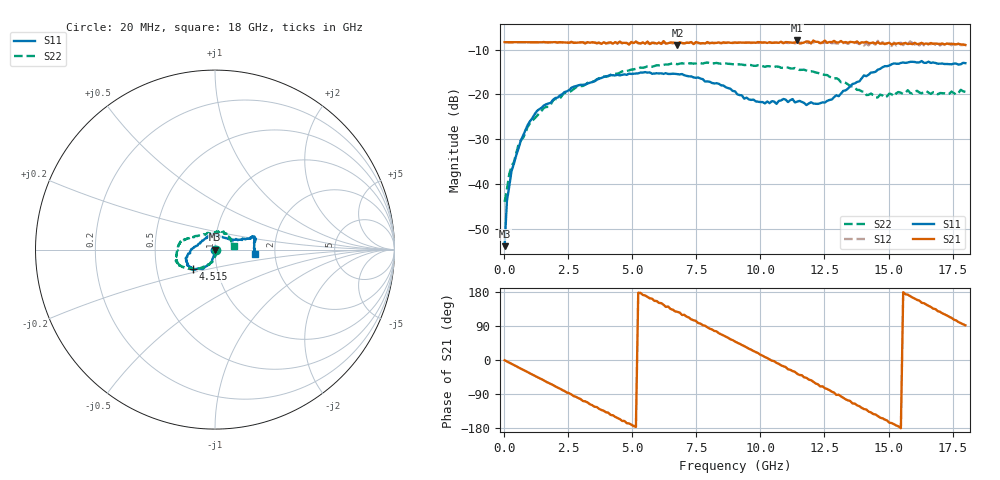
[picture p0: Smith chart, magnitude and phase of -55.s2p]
!Agilent Technologies,N5230A,US43500223,A.07.50.48
!Agilent N5230A: A.07.50.48
!Date: Monday, February 01, 2016 14:55:05
!Correction: S11(Full 2 Port(1,2))
!S21(Full 2 Port(1,2))
!S12(Full 2 Port(1,2))
!S22(Full 2 Port(1,2))
!S2P File: Measurements: S11, S21, S12, S22:
# Hz S  RI  R 50
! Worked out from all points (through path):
!   201 points, 20 MHz to 18 GHz, reference 50 ohm
!   highest |S21| = -7.93 dB at 11.44 GHz (marker M1); lowest = -9.0 dB at 6.763 GHz (marker M2)
!   group delay of S21, straight-line fit = 96.8 ps
!   lowest |S11| = -53.9 dB at 20 MHz (marker M3), VSWR 1.00, Z = 49.8 - j0.107 ohm
!   |S11| at or under -10 dB: start of sweep to end of sweep
!   |S22| runs from -44.0 to -12.9 dB; largest |S21 - S12| = 0.035
!   S11 on the Smith chart (normalised r, x): 20 MHz: 1.00, -0.00; 4.515 GHz: 0.76, -0.17; 18 GHz: 1.57, -0.08
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2e7  -0.00171 -0.00107  0.3841 -0.00414  0.3835 -0.00465  0.0063 -0.00049
1.099e8  0.000891 -0.00637  0.3827 -0.0255  0.382 -0.0262  0.00665 -0.00559
2.897e8  0.00118 -0.0139  0.3777 -0.0676  0.3772 -0.0679  0.00786 -0.0138
9.19e8  -0.00995 -0.0444  0.3258 -0.2035  0.3246 -0.2048  -0.00213 -0.0434
1.5483e9  -0.0198 -0.0726  0.2279 -0.3103  0.2256 -0.3116  -0.0149 -0.069
3.0766e9  -0.0713 -0.1064  -0.1199 -0.3631  -0.118 -0.364  -0.0748 -0.0994
4.515e9  -0.1236 -0.1068  -0.3538 -0.1585  -0.3572 -0.1582  -0.1406 -0.1042
6.0433e9  -0.1579 -0.067  -0.331 0.1856  -0.323 0.1978  -0.1912 -0.0904
6.7625e9  -0.1615 -0.0482  -0.2143 0.2825  -0.2117 0.2962  -0.2018 -0.0817
7.9312e9  -0.1393 -0.013  0.0249 0.384  0.0334 0.3739  -0.2188 -0.0623
9.01e9  -0.1066 0.0201  0.2512 0.287  0.2574 0.2757  -0.2151 -0.0311
1.00888e10  -0.0551 0.061  0.3727 0.0747  0.375 0.0612  -0.207 0.00587
1.14373e10  -0.00286 0.083  0.3227 -0.2384  0.2992 -0.234  -0.1866 0.0462
1.20666e10  0.0269 0.0745  0.2152 -0.3382  0.1857 -0.3356  -0.1699 0.0586
1.27858e10  0.0594 0.0647  0.0438 -0.3814  0.0167 -0.3729  -0.1383 0.0671
1.3505e10  0.1107 0.0545  -0.121 -0.3684  -0.1441 -0.3508  -0.098 0.075
1.44939e10  0.17 0.0571  -0.2981 -0.2179  -0.2896 -0.2139  -0.0259 0.089
1.50333e10  0.1992 0.067  -0.3654 -0.0948  -0.3544 -0.0746  0.00981 0.102
1.58424e10  0.2195 0.0728  -0.3631 0.0726  -0.3808 0.0935  0.0523 0.0901
1.64717e10  0.2199 0.0502  -0.3094 0.2055  -0.3091 0.2143  0.0745 0.0801
1.73707e10  0.2176 0.012  -0.1483 0.3338  -0.1217 0.3517  0.0898 0.0478
1.8e10  0.2226 -0.0233  -0.0096 0.3568  0.025 0.3578  0.1052 0.0199
